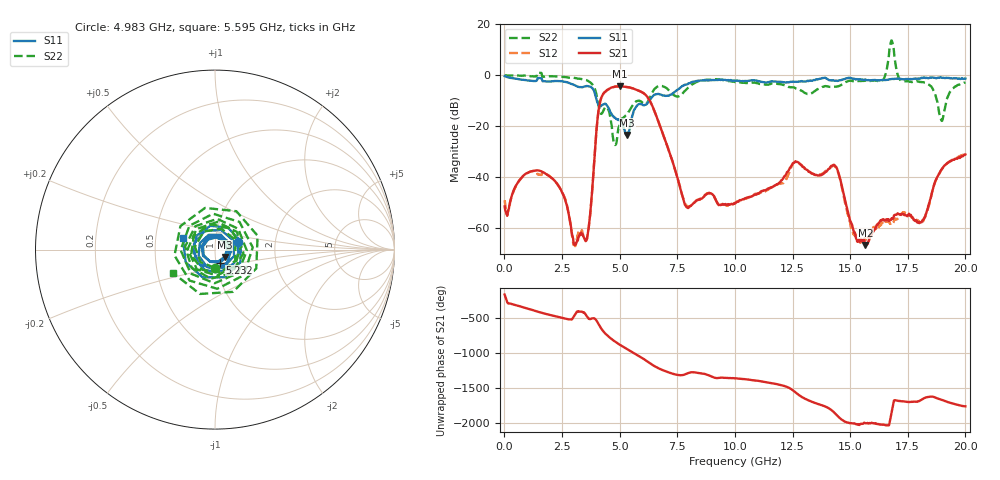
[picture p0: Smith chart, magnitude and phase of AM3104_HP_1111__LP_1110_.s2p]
!Created with skrf (http://scikit-rf.org).
# Hz S RI R 50.0
!freq ReS11 ImS11 ReS21 ImS21 ReS12 ImS12 ReS22 ImS22
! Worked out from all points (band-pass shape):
!   1601 points, 10 MHz to 20 GHz, reference 50 ohm
!   highest |S21| = -4.37 dB at 4.995 GHz (marker M1); lowest = -66.5 dB at 15.66 GHz (marker M2)
!   |S21| within 3 dB of the highest: 4.286 GHz to 6.088 GHz (1.803 GHz wide, 34.8 % of centre)
!   lowest |S11| = -23.4 dB at 5.332 GHz (marker M3), VSWR 1.14, Z = 55.5 - j4.5 ohm
!   |S11| at or under -10 dB: 4.013 GHz to 6.292 GHz (2.279 GHz wide, 44.2 % of centre)
!   |S22| runs from -27.3 to 13.6 dB; largest |S21 - S12| = 0.072
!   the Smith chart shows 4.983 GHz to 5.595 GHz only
!   S11 on the Smith chart (normalised r, x): 4.983 GHz: 1.29, +0.11; 5.232 GHz: 1.05, -0.15; 5.595 GHz: 0.69, +0.09
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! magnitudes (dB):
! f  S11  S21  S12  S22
! 10 MHz  -0.4  -51.4  -49.0  0.0
! 1.572 GHz  -1.2  -37.5  -39.1  0.9
! 3.033 GHz  -3.8  -66.3  -66.6  -1.0
! 3.346 GHz  -4.7  -61.9  -61.1  -1.5
! 3.658 GHz  -4.4  -59.8  -59.5  -2.4
! 4.17 GHz  -12.2  -9.7  -9.8  -14.8
! 4.983 GHz  -17.5  -4.4  -4.4  -19.9
! 4.995 GHz  -17.6  -4.4  -4.4  -19.4
! 5.232 GHz  -22.3  -4.5  -4.5  -16.1
! 5.332 GHz  -23.4  -4.6  -4.6  -15.2
! 5.595 GHz  -14.5  -5.2  -5.2  -11.5
! 6.682 GHz  -7.3  -18.1  -18.2  -4.3
! 7.894 GHz  -3.7  -51.6  -51.1  -5.6
! 10.01 GHz  -2.2  -50.3  -50.0  -2.7
! 13.34 GHz  -2.2  -38.5  -38.5  -7.0
! 14.37 GHz  -2.1  -35.7  -36.0  -4.5
! 15.13 GHz  -1.4  -60.2  -61.8  -2.3
! 15.66 GHz  -1.7  -66.5  -64.3  -2.1
! 16.68 GHz  -1.6  -56.7  -57.4  7.3
! 18.1 GHz  -1.0  -57.6  -57.8  -2.7
! 18.96 GHz  -1.0  -36.9  -37.0  -17.7
! 20 GHz  -1.3  -31.0  -30.8  -2.9
